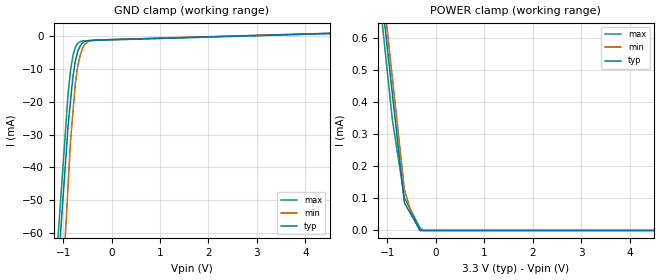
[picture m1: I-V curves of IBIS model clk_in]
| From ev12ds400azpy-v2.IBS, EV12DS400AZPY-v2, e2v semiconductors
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[Model] clk_in
Model_type Input
Vinl = 2.20000V
Vinh = 2.80000V
C_comp 569.000fF 560.000fF 578.000fF
| variable typ   min   max
[Voltage Range] 3.30000V 3.15000V 3.45000V
[POWER Clamp Reference] 3.30000V 3.15000V 3.45000V
[GND Clamp Reference] 0.00000V 0.00000V 0.00000V
[Temperature Range]   25   110   -40
[GND Clamp]
-3.3V     -535mA     -693.2mA   -525.4mA
-900mV    -27.39mA   -45.62mA   -17.6mA
-850mV    -19.9mA    -32.13mA   -10.56mA
-800mV    -12.4mA    -23.26mA   -5.964mA
-750mV    -7.602mA   -14.4mA    -3.366mA
-700mV    -4.59mA    -9.025mA   -2.127mA
-650mV    -2.984mA   -5.811mA   -1.629mA
-600mV    -2.014mA   -3.617mA   -1.41mA
-550mV    -1.542mA   -2.378mA   -1.377mA
-500mV    -1.333mA   -1.723mA   -1.345mA
-400mV    -1.253mA   -1.214mA   -1.28mA
6.6V      1.781mA    1.816mA    1.733mA
[POWER Clamp]
-3.3V     3.727mA    3.855mA    3.822mA
-900mV    430.2uA    480.1uA    348.5uA
-650mV    86.78uA    128.6uA    102.2uA
-500mV    46.73uA    51.44uA    58.39uA
-450mV    33.38uA    36.74uA    43.79uA
-325mV    0A         0A         7.298uA
-250mV    0A         0A         0A
6.6V      0A         0A         0A
